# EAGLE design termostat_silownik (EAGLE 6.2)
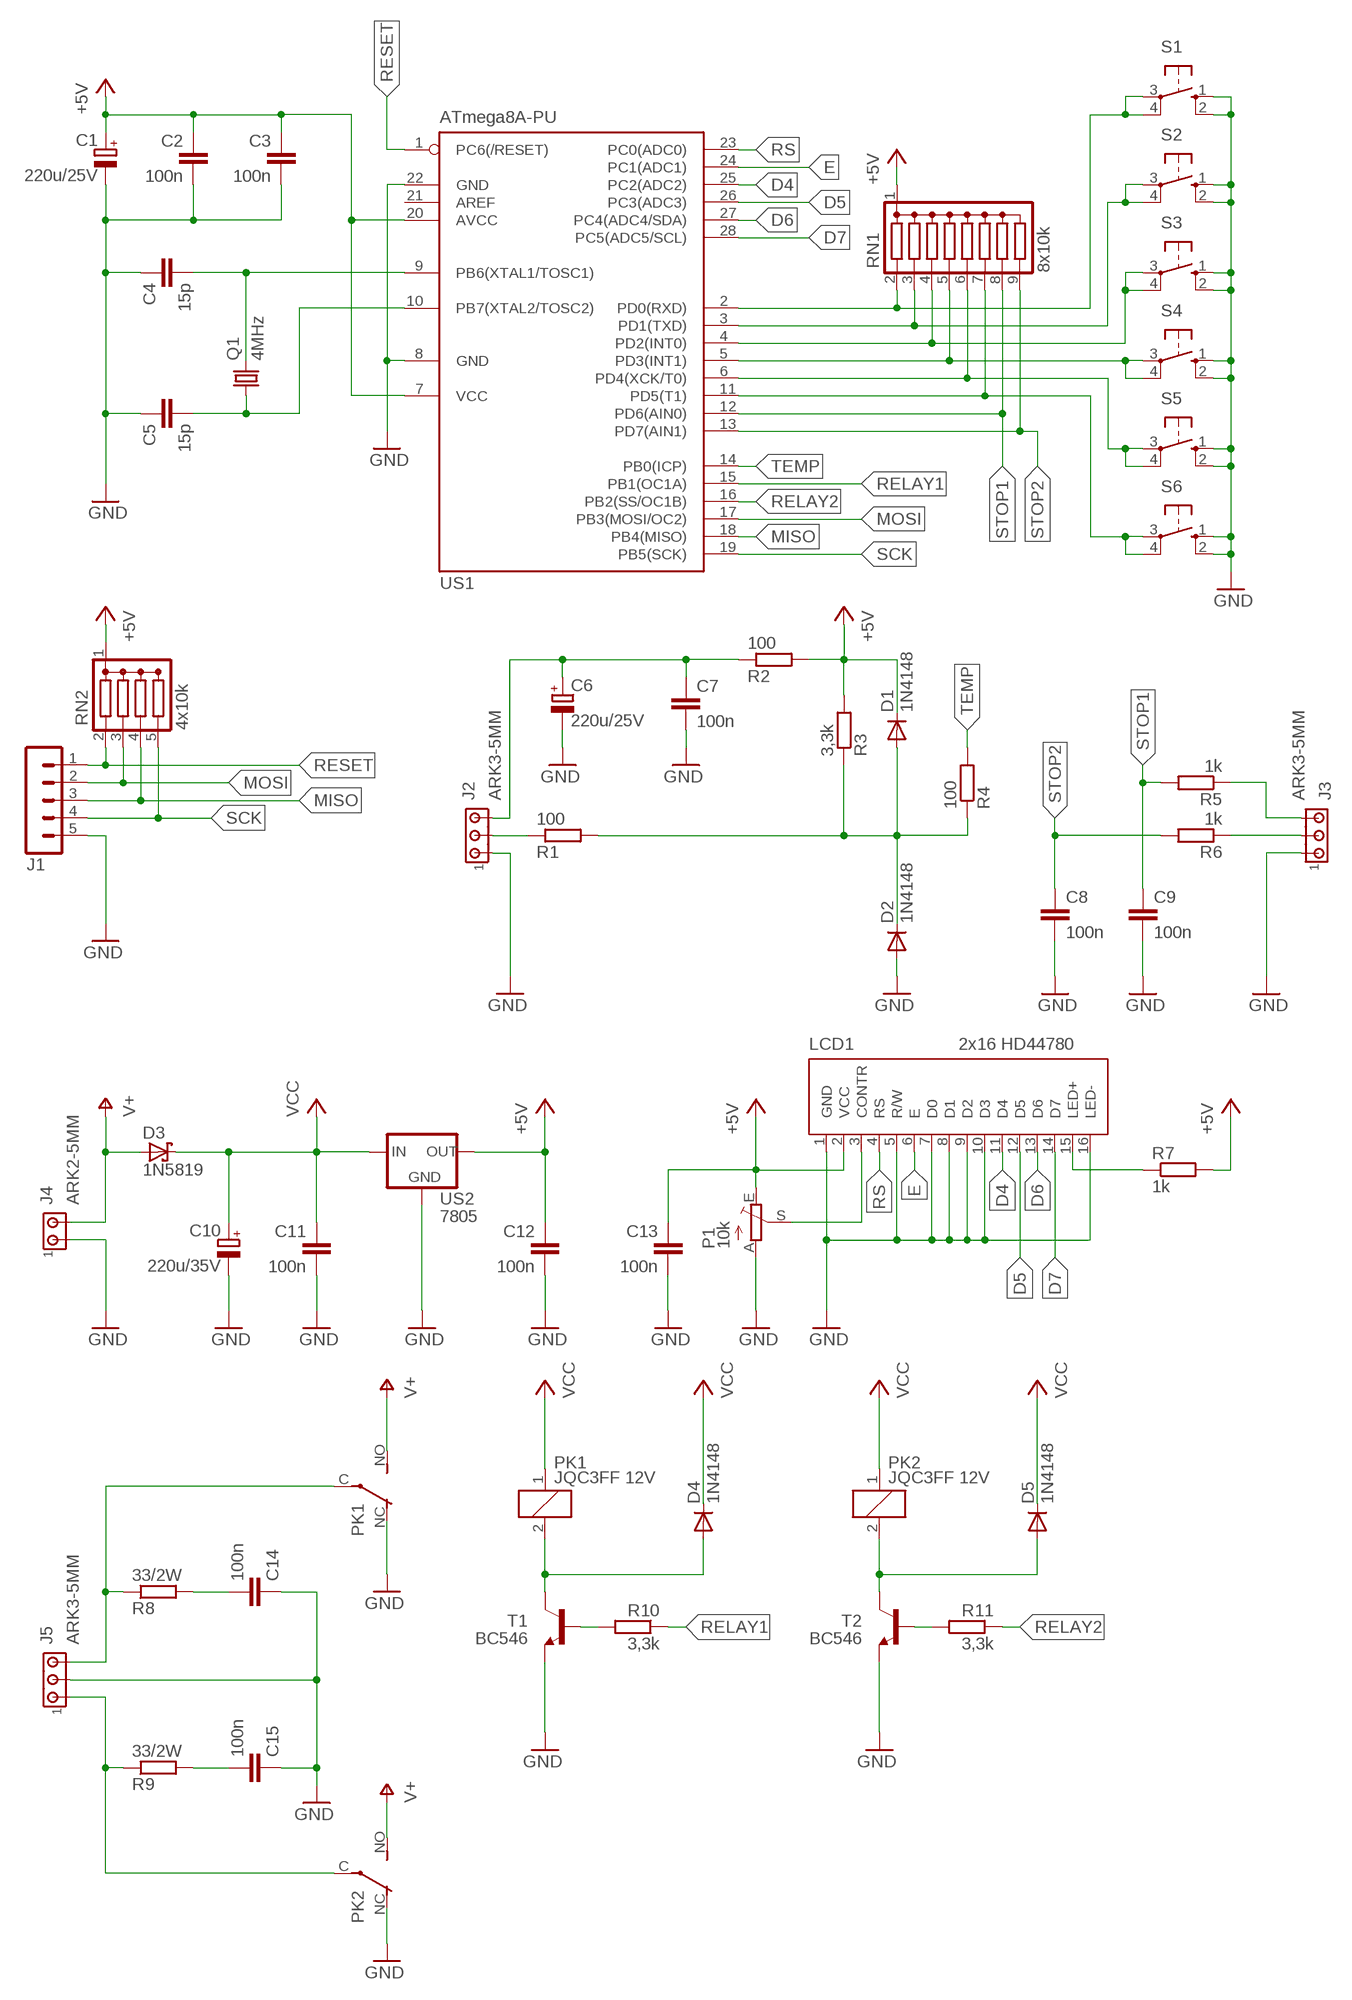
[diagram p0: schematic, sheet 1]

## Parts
C1  220u/25V  CPOL-EUE2.5-7  [E2,5-7]
C2  100n  C-EU050-025X075  [C050-025X075]
C3  100n  C-EU050-025X075  [C050-025X075]
C4  15p  C-EU050-025X075  [C050-025X075]
C5  15p  C-EU050-025X075  [C050-025X075]
C6  220u/25V  CPOL-EUE2.5-7  [E2,5-7]
C7  100n  C-EU050-025X075  [C050-025X075]
C8  100n  C-EU050-025X075  [C050-025X075]
C9  100n  C-EU050-025X075  [C050-025X075]
C10  220u/35V  CPOL-EUE3.5-8  [E3,5-8]
C11  100n  C-EU050-025X075  [C050-025X075]
C12  100n  C-EU050-025X075  [C050-025X075]
C13  100n  C-EU050-025X075  [C050-025X075]
C14  100n  C-EU050-025X075  [C050-025X075]
C15  100n  C-EU050-025X075  [C050-025X075]
D1  1N4148  BAT81  [DO34-7]
D2  1N4148  BAT81  [DO34-7]
D3  1N5819  SCHOTTKY-DIODEF126Z12  [F126Z12]
D4  1N4148  BAT81  [DO34-7]
D5  1N4148  BAT81  [DO34-7]
J1  MA05-1  [MA05-1]
J2  ARK3-5MM  [3PIN-5MM]
J3  ARK3-5MM  [3PIN-5MM]
J4  ARK2-5MM  [2PIN-5MM]
J5  ARK3-5MM  [3PIN-5MM]
LCD1  2x16 HD44780  LCD_2X16-NAD-ELEMENTAMI  [LCD_HD44780_2X16_NAD-ELEMENTAMI]
P1  10k  TRIM_EU-CA6V  [CA6V]
PK1  JQC3FF 12V  PK_POJED-JQC-3FG  [PK_POJED_JQC-3FG]
PK2  JQC3FF 12V  PK_POJED-JQC-3FG  [PK_POJED_JQC-3FG]
Q1  4MHz  CRYSTALHC49U-V  [HC49U-V]
R1  100  R-EU_0207/7  [0207/7]
R2  100  R-EU_0207/7  [0207/7]
R3  3,3k  R-EU_0207/7  [0207/7]
R4  100  R-EU_0207/7  [0207/7]
R5  1k  R-EU_0207/7  [0207/7]
R6  1k  R-EU_0207/7  [0207/7]
R7  1k  R-EU_0207/7  [0207/7]
R8  33/2W  R-EU_0411/15  [0411/15]
R9  33/2W  R-EU_0411/15  [0411/15]
R10  3,3k  R-EU_0207/7  [0207/7]
R11  3,3k  R-EU_0207/7  [0207/7]
RN1  8x10k  DRAB_REZ_1X8-SIL9  [RN-9]
RN2  4x10k  DRAB_REZ_1X4  [RN-5]
S1  10-XX  [B3F-10XX]
S2  10-XX  [B3F-10XX]
S3  10-XX  [B3F-10XX]
S4  10-XX  [B3F-10XX]
S5  10-XX  [B3F-10XX]
S6  10-XX  [B3F-10XX]
T1  BC546  BC546A  [TO92-EBC]
T2  BC546  BC546A  [TO92-EBC]
US1  ATmega8A-PU  MEGA8-P  [DIL28-3]
US2  7805  78XXS  [78XXS]

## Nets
+5V: C1.+ C2.1 C3.1 C12.1 C13.1 D1.C LCD1.2(VCC) P1.E R2.2 R3.2 R7.2 RN1.1(C) RN2.1(C) US1.7(VCC) US1.20(AVCC) US2.OUT
D4: LCD1.11(D4) US1.25(PC2(ADC2))
D5: LCD1.12(D5) US1.26(PC3(ADC3))
D6: LCD1.13(D6) US1.27(PC4(ADC4/SDA))
D7: LCD1.14(D7) US1.28(PC5(ADC5/SCL))
E: LCD1.6(E) US1.24(PC1(ADC1))
GND: C1.- C2.2 C3.2 C4.1 C5.1 C6.- C7.2 C8.2 C9.2 C10.- C11.2 C12.2 C13.2 C14.1 C15.1 D2.A J1.5 J2.P$1 J3.P$1 J4.P$1 J5.P$2 LCD1.1(GND) LCD1.5(R/W) LCD1.7(D0) LCD1.8(D1) LCD1.9(D2) LCD1.10(D3) LCD1.16(LED-) P1.A PK1.NC PK2.NC S1.1(S) S1.2(S1) S2.1(S) S2.2(S1) S3.1(S) S3.2(S1) S4.1(S) S4.2(S1) S5.1(S) S5.2(S1) S6.1(S) S6.2(S1) T1.E T2.E US1.8(GND) US1.22(GND) US2.GND
MISO: J1.3 RN2.4 US1.18(PB4(MISO))
MOSI: J1.2 RN2.3 US1.17(PB3(MOSI/OC2))
N$1: LCD1.3(CONTR) P1.S
N$2: R11.2 T2.B
N$3: C5.2 Q1.1 US1.10(PB7(XTAL2/TOSC2))
N$4: C4.2 Q1.2 US1.9(PB6(XTAL1/TOSC1))
N$5: RN1.2 S1.3(P) S1.4(P1) US1.2(PD0(RXD))
N$6: LCD1.15(LED+) R7.1
N$7: R10.2 T1.B
N$8: C15.2 R9.2
N$9: D4.A PK1.2 T1.C
N$10: RN1.3 S2.3(P) S2.4(P1) US1.3(PD1(TXD))
N$11: D5.A PK2.2 T2.C
N$12: C14.2 R8.2
N$13: RN1.4 S3.3(P) S3.4(P1) US1.4(PD2(INT0))
N$14: RN1.5 S4.3(P) S4.4(P1) US1.5(PD3(INT1))
N$15: RN1.6 S5.3(P) S5.4(P1) US1.6(PD4(XCK/T0))
N$16: RN1.7 S6.3(P) S6.4(P1) US1.11(PD5(T1))
N$17: J5.P$1 PK2.C(COM) R9.1
N$18: J5.P$3 PK1.C(COM) R8.1
N$19: C6.+ C7.1 J2.P$3 R2.1
N$20: J2.P$2 R1.1
N$21: D1.A D2.C R1.2 R3.1 R4.1
N$25: J3.P$2 R6.1
N$26: J3.P$3 R5.1
RELAY1: R10.1 US1.15(PB1(OC1A))
RELAY2: R11.1 US1.16(PB2(SS/OC1B))
RESET: J1.1 RN2.2 US1.1(PC6(/RESET))
RS: LCD1.4(RS) US1.23(PC0(ADC0))
SCK: J1.4 RN2.5 US1.19(PB5(SCK))
STOP1: C9.1 R5.2 RN1.8 US1.12(PD6(AIN0))
STOP2: C8.1 R6.2 RN1.9 US1.13(PD7(AIN1))
TEMP: R4.2 US1.14(PB0(ICP))
V+: D3.A J4.P$2 PK1.NO PK2.NO
VCC: C10.+ C11.1 D3.C D4.C D5.C PK1.1 PK2.1 US2.IN
Unconnected: US1.21(AREF)

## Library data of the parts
C1 C6 C10 = rcl:CPOL-EU: POLARIZED CAPACITOR, European symbol
C2-C5 C7-C9 C11-C15 = rcl:C-EU: CAPACITOR, European symbol
D1 D2 D4 D5 = diode:BAT81: DIODE
D3 = diode:SCHOTTKY-DIODE: Schottky Diode
J1 = zlacza_futrzak:MA05-1: PIN HEADER; OC_FARNELL: unknown; OC_NEWARK: unknown
J2 J3 J5 = zlacza_futrzak:ARK3: ARK 3 Raster 5mm i 3,5mm
J4 = zlacza_futrzak:ARK2: ARK 2
LCD1 = inne_futrzak:LCD_2X16
P1 = pot:TRIM_EU-: POTENTIOMETER
PK1 PK2 = inne_futrzak:PK_POJED
Q1 = crystal:CRYSTAL: CRYSTAL; OC_FARNELL: 1666969; OC_NEWARK: unknown
R1-R11 = rcl:R-EU_: RESISTOR, European symbol
RN1 = inne_futrzak:DRAB_REZ_1X8
RN2 = inne_futrzak:DRAB_REZ_1X4
S1-S6 = switch-omron:10-XX: OMRON SWITCH; MPN: B3F-1000; OC_FARNELL: 176432; OC_NEWARK: 36M3542
T1 T2 = transistor-npn:BC546*: NPN Transistor
US1 = atmel:MEGA8-P: MICROCONTROLLER 8 Kbytes FLASH, 1 kbytes SRAM, 512 bytes EEPROM, USART, 4-channel 10 bit ADC, 2-channel 8 bit ADC Pin compatible with Atmega48, ATMega88, ATMega168 Source: avr.lbr; OC_FARNELL: unknown; OC_NEWARK: unknown
US2 = v-reg:78XXS: VOLTAGE REGULATOR

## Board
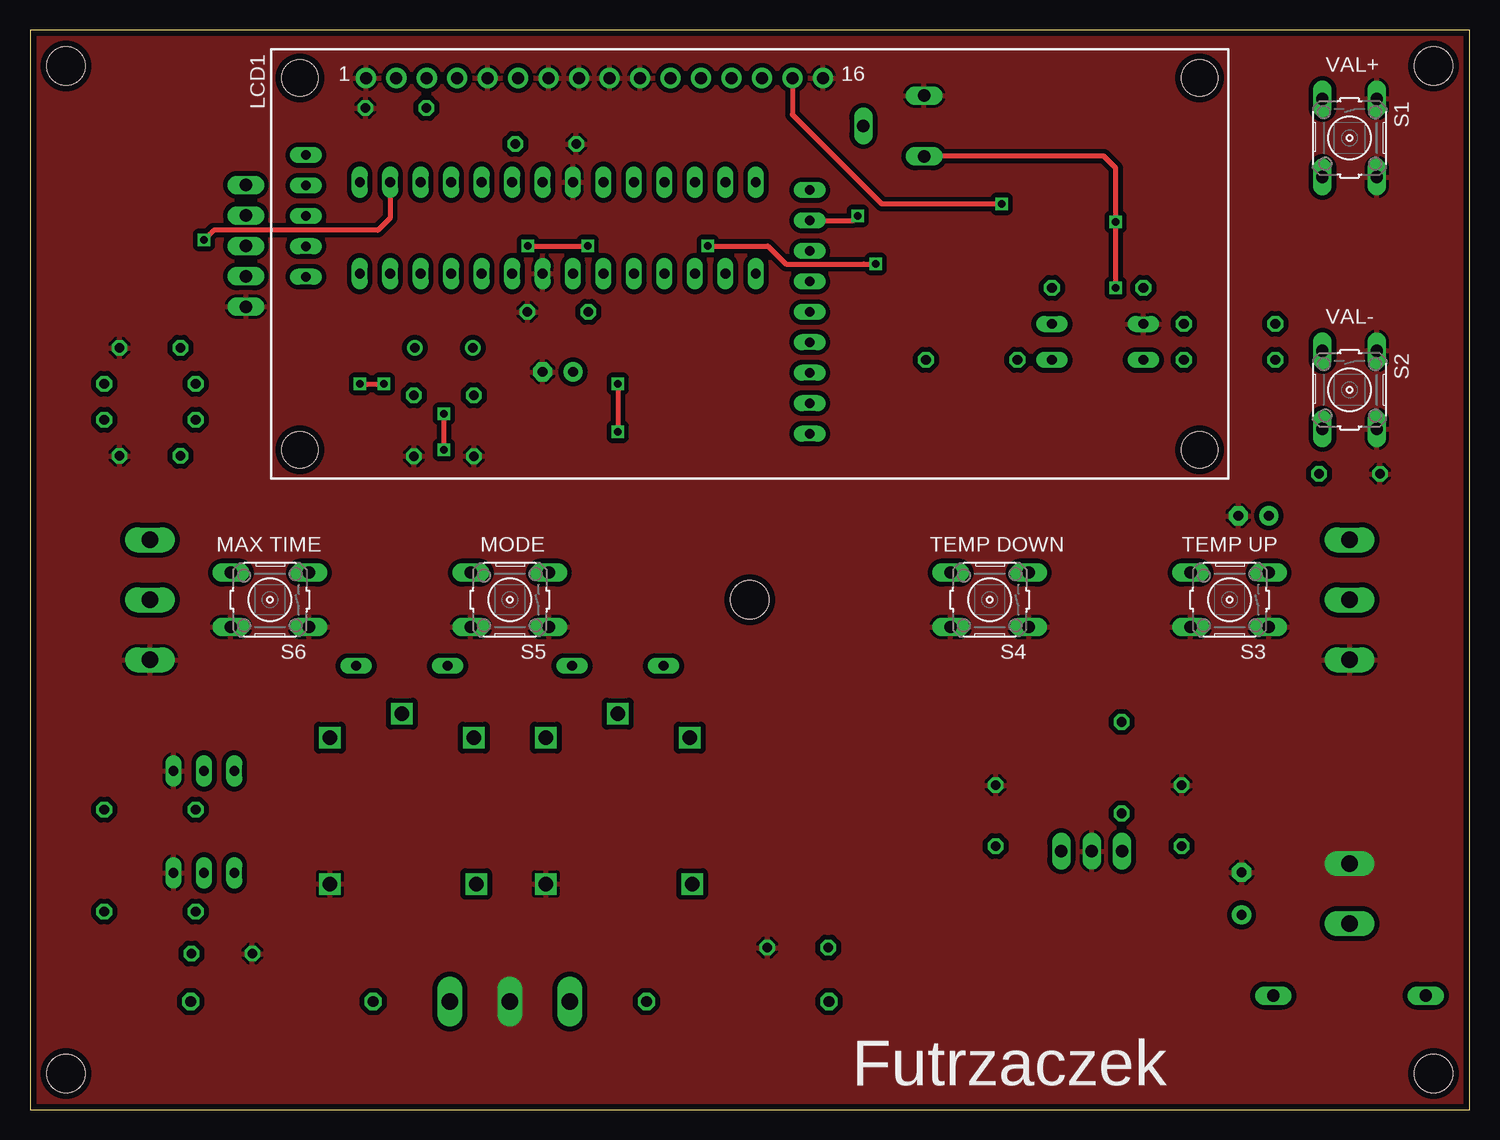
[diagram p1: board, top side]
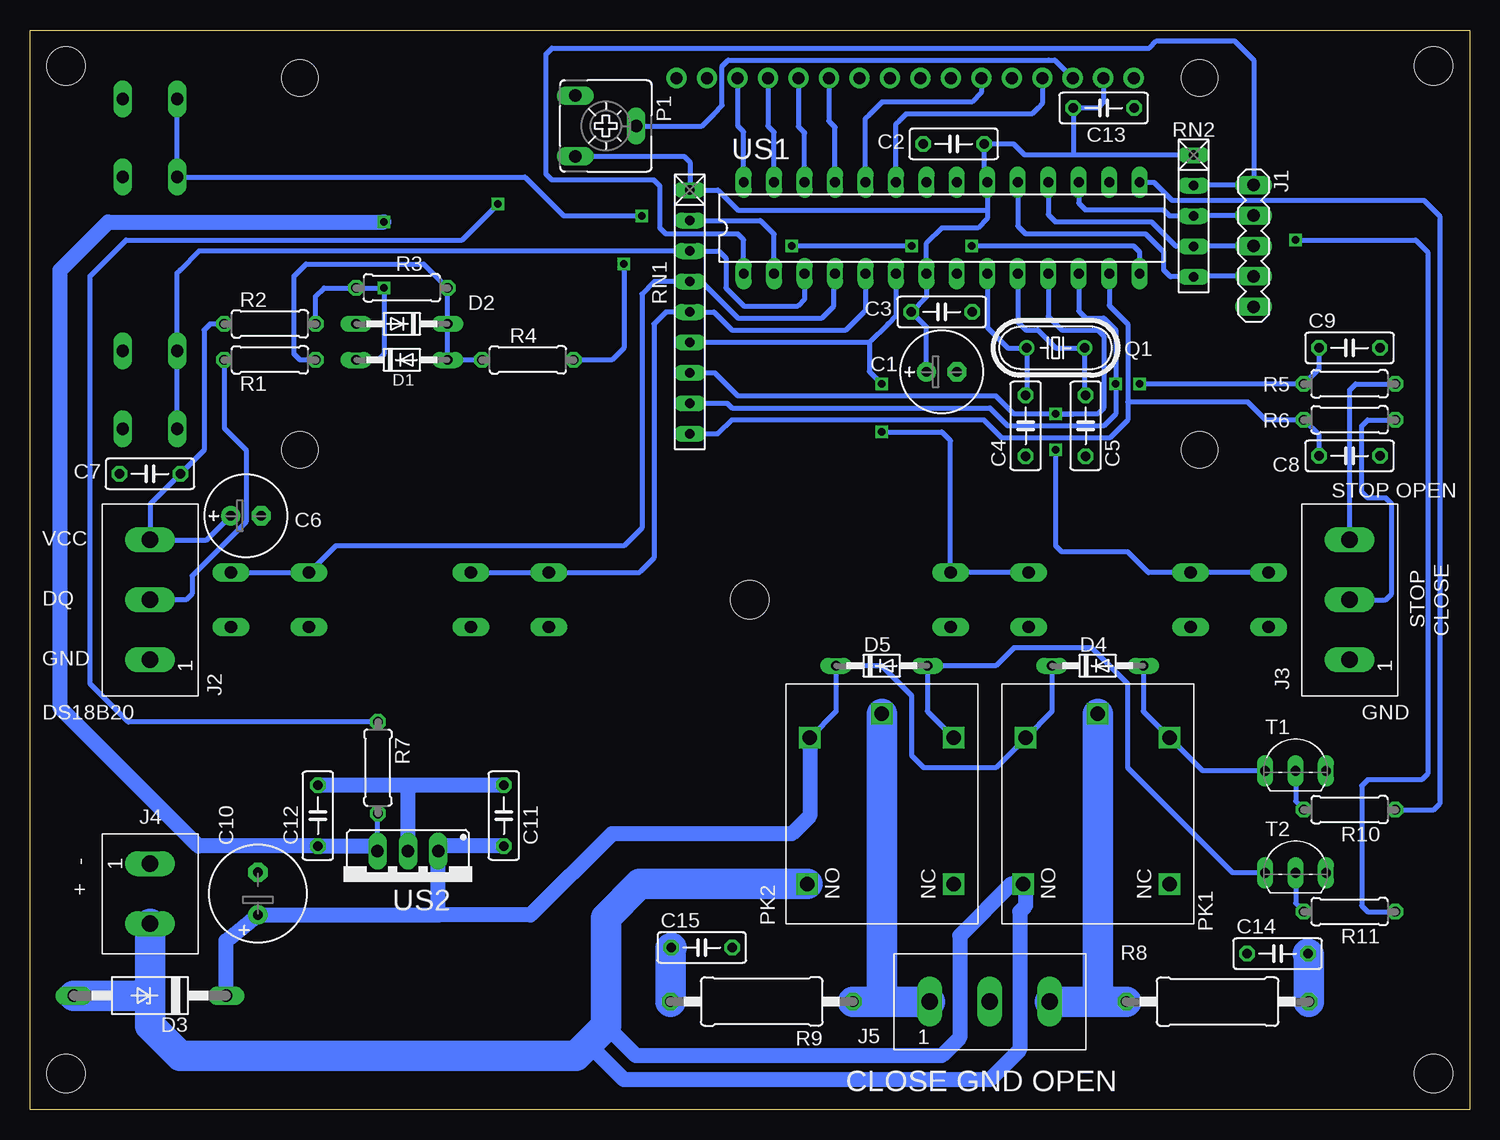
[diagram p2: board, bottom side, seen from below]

Size 120 x 90 mm. Coordinates in mm from the lower left corner, seen from the top.
Outline: 0,0 120,0 120,90 0,90 0,0
Copper layers (1*16): Top 0.035mm / dielectric 1.5mm / Bottom 0.035mm
Design rules: minimum track width 10mil, minimum drill 23mil, track to track 8mil, track to pad 8mil, pad to pad 8mil, via to via 8mil, smd to smd 8mil, copper to edge 20mil, drill to drill 8mil, minimum pad ring 10mil, minimum via ring 8mil, stop-mask expansion 4mil, vias tented up to drill 0mil, thermal gap 10mil
Holes 3.2 mm at 3,87 117,87 3,3 117,3 60,42.5

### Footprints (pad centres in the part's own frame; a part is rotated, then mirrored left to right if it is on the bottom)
E2,5-7 = drill 0.813 pad 1.6: + -1.27,0 | drill 0.813 pad 1.6 octagon: - 1.27,0
C050-025X075 = drill 0.813 octagon: 1 -2.54,0; 2 2.54,0
E3,5-8 = drill 0.813 pad 1.6: + -1.778,0 | drill 0.813 pad 1.6 octagon: - 1.778,0
DO34-7 = drill 0.813 long: A 3.81,0; C -3.81,0
F126Z12 = drill 1.016 long: A 6.35,0; C -6.35,0
MA05-1 = drill 1.016 long: 1 -5.08,0; 2 -2.54,0; 3 0,0; 4 2.54,0; 5 5.08,0
3PIN-5MM = drill 1.4 long: P$1 -5,0; P$2 0,0; P$3 5,0
2PIN-5MM = drill 1.4 long: P$1 -2.5,0; P$2 2.5,0
LCD_HD44780_2X16_NAD-ELEMENTAMI = drill 1 pad 1.676: 1 -32,15.5; 2 -29.46,15.5; 3 -26.92,15.5; 4 -24.38,15.5; 5 -21.84,15.5; 6 -19.3,15.5; 7 -16.76,15.5; 8 -14.22,15.5; 9 -11.68,15.5; 10 -9.14,15.5; 11 -6.6,15.5; 12 -4.06,15.5; 13 -1.52,15.5; 14 1.02,15.5; 15 3.56,15.5; 16 6.1,15.5 | hole 3: -37.5,-15.5; 37.5,-15.5; -37.5,15.5; 37.5,15.5
CA6V = drill 1.016 long: A -2.54,-2.54; E 2.54,-2.54; S 0,2.54
PK_POJED_JQC-3FG = drill 1.2 square: 1 5.5,6; 2 5.5,-6; C 7.5,0; NC -6.7,-6; NO -6.7,6.2
HC49U-V = drill 0.813: 1 -2.413,0; 2 2.413,0
0207/7 = drill 0.813 octagon: 1 -3.81,0; 2 3.81,0
0411/15 = drill 0.914 octagon: 1 -7.62,0; 2 7.62,0
RN-9 = drill 0.813 long: 1 -10.16,0; 2 -7.62,0; 3 -5.08,0; 4 -2.54,0; 5 0,0; 6 2.54,0; 7 5.08,0; 8 7.62,0; 9 10.16,0
RN-5 = drill 0.813 long: 1 -5.08,0; 2 -2.54,0; 3 0,0; 4 2.54,0; 5 5.08,0
B3F-10XX = drill 1.016 long: 1 -3.251,2.261; 2 3.251,2.261; 3 -3.251,-2.261; 4 3.251,-2.261
TO92-EBC = drill 0.813 long: B 0,-1.27; C -2.54,-1.27; E 2.54,-1.27
DIL28-3 = drill 0.813 long: 1 -16.51,-3.81; 2 -13.97,-3.81; 3 -11.43,-3.81; 4 -8.89,-3.81; 5 -6.35,-3.81; 6 -3.81,-3.81; 7 -1.27,-3.81; 8 1.27,-3.81; 9 3.81,-3.81; 10 6.35,-3.81; 11 8.89,-3.81; 12 11.43,-3.81; 13 13.97,-3.81; 14 16.51,-3.81; 15 16.51,3.81; 16 13.97,3.81; 17 11.43,3.81; 18 8.89,3.81; 19 6.35,3.81; 20 3.81,3.81; 21 1.27,3.81; 22 -1.27,3.81; 23 -3.81,3.81; 24 -6.35,3.81; 25 -8.89,3.81; 26 -11.43,3.81; 27 -13.97,3.81; 28 -16.51,3.81
78XXS = drill 1.016 long: GND 0,-2.54; IN -2.54,-2.54; OUT 2.54,-2.54

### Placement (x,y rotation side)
C1  44,61.5 0 bottom
C2  43,80.5 180 bottom
C3  44,66.5 0 bottom
C4  37,57 90 bottom
C5  32,57 90 bottom
C6  102,49.5 0 bottom
C7  110,53 180 bottom
C8  10,54.5 0 bottom
C9  10,63.5 0 bottom
C10  101,18 90 bottom
C11  80.5,24.5 90 bottom
C12  96,24.5 90 bottom
C13  30.5,83.5 0 bottom
C14  16,13 0 bottom
C15  64,13.5 180 bottom
D1  89,62.5 0 bottom
D2  89,65.5 180 bottom
D3  110,9.5 180 bottom
D4  31,37 0 bottom
D5  49,37 0 bottom
J1  18,72 270 bottom
J2  110,42.5 90 bottom
J3  10,42.5 90 bottom
J4  110,18 270 bottom
J5  40,9 0 bottom
LCD1  60,70.5 0 top
P1  72,82 270 bottom
PK1  31,25.5 90 bottom
PK2  49,25.5 90 bottom
Q1  34.5,63.5 180 bottom
R1  100,62.5 0 bottom
R2  100,65.5 0 bottom
R3  89,68.5 180 bottom
R4  78.5,62.5 0 bottom
R5  10,60.5 180 bottom
R6  10,57.5 180 bottom
R7  91,28.5 270 bottom
R8  21,9 0 bottom
R9  59,9 180 bottom
R10  10,25 180 bottom
R11  10,16.5 180 bottom
RN1  65,66.5 270 bottom
RN2  23,74.5 270 bottom
S1  110,81 270 top
S2  110,60 270 top
S3  100,42.5 180 top
S4  80,42.5 180 top
S5  40,42.5 180 top
S6  20,42.5 180 top
T1  14.5,29.5 0 bottom
T2  14.5,21 0 bottom
US1  44,73.5 0 bottom
US2  88.5,19 180 bottom

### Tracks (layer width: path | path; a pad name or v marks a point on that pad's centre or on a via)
+5V  (via drill 0.6)
  Top 0.406: v90.5,68.5 v90.5,74 90.5,78.5 89.5,79.5 74.58,79.5 P1.E
  Bottom 0.406: 40.19,75 US1.20 40.46,77.58 C2.1 38,80.5 37.08,79.58 33,79.58 | 40.19,75 40.19,74.31 41,73.5 44,73.5 45.27,72.23 US1.7 45.27,67.77 C3.1 45.27,65.23 C1.+ | RN2.1 33,79.58 | 33,79.58 33.04,79.62 C13.1 31,83.5 30.54,83.96 LCD1.2 | 40.19,75 61,75 62.66,76.66 RN1.1 65,79 65.46,79.46 P1.E | D1.C 91,62.5 90.5,63 v90.5,68.5 R3.2 95.5,68.5 96.19,67.81 R2.2 | US2.OUT 91.04,24.65 R7.2
  Bottom 1.27: v90.5,74 113.5,74 117.5,70 117.5,33.5 105.96,21.96 C12.1 91.04,21.96 US2.OUT
D4
  Bottom 0.406: US1.25 52.89,81.89 53,82 53.4,82.4 LCD1.11
D5
  Bottom 0.406: US1.26 55.43,81.43 55.94,81.94 LCD1.12
D6
  Bottom 0.406: US1.27 57.97,81.47 58.48,81.98 LCD1.13
D7
  Bottom 0.406: US1.28 60.51,81.51 61,82 61.02,82.02 LCD1.14
E
  Bottom 0.406: LCD1.6 40.7,84.8 41.5,84 49,84 50,83 50.35,82.65 US1.24
GND
  Bottom 1.27: C11.2 88.5,27.04 | 88.5,27.04 C12.2 | US2.GND 88.5,27.04
  pour Top (isolate 0.406): 0,0 120,0 120,90 0,90
  pour Top (no thermals): 38.5,12 41.5,12 41.5,6 38.5,6
  pour Top (no thermals): 107.5,22 112.5,22 112.5,19 107.5,19
MISO
  Bottom 0.406: J1.3 22.96,72 RN2.4 24.46,71.96 26.5,74 34.5,74 35.11,74.61 US1.18
MOSI
  Bottom 0.406: J1.2 22.96,74.54 RN2.3 25,74.5 25.5,75 32,75 32.57,75.57 US1.17
N$1
  Bottom 0.406: P1.S 64,82 63,83 62.3,83.7 62.3,87 61.8,87.5 35.08,87.5 34.58,87.5 LCD1.3
N$2
  Bottom 0.406: T2.B 14.5,17.19 R11.2
N$3
  Bottom 0.406: US1.10 37.65,65.65 37,65 36,65 34.5,63.5 Q1.1 32.09,59.63 C5.2
N$4
  Bottom 0.406: US1.9 40.19,65.19 38.5,63.5 Q1.2 36.91,59.63 C4.2
N$5  (via drill 0.6)
  Top 0.406: RN1.2 68.62,74.12 v69,74.5
  Bottom 0.406: RN1.2 59.12,74.12 58,73 57.97,72.97 US1.2 | v69,74.5 75.5,74.5 78.5,77.5 78.75,77.75 S1.4 S1.3
N$6  (via drill 0.6)
  Top 0.406: v81,75.5 71,75.5 63.56,82.94 LCD1.15
  Bottom 0.406: R7.1 111.81,32.31 115,35.5 115,69.5 112,72.5 84,72.5 v81,75.5
N$7
  Bottom 0.406: T1.B 14.5,25.69 R10.2
N$8
  Bottom 2.54: R9.2 66.62,13.42 C15.2
N$9
  Bottom 0.406: T1.C 22.23,28.23 PK1.2 27.19,33.19 D4.A
N$10
  Bottom 0.406: US1.3 55.43,67.57 56,67 60.5,67 62,68.5 62,71 62.58,71.58 RN1.3 105.92,71.58 107.5,70 107.74,69.76 S2.3 S2.4
N$11
  Bottom 0.406: PK2.2 45.19,33.19 D5.A 39.5,37 38,38.5 31.5,38.5 28.5,35.5 28.5,28.5 19.73,19.73 T2.C
N$12
  Bottom 2.54: R8.2 13.38,12.92 C14.2
N$13
  Bottom 0.406: US1.4 53,69.58 53,67 54,66 61,66 63,68 64.04,69.04 RN1.4 67.96,69.04 69,68 69,48.5 70.5,47 94.51,47 S3.4 S3.3
N$14
  Bottom 0.406: US1.5 50.35,66.65 50.5,66.5 52,65 61.5,65 63,66.5 RN1.5 67,66.5 68,65.5 68,46 69,45 69.24,44.76 S4.4 S4.3
N$15  (via drill 0.6)
  Top 0.406: v49,60.5 v49,56.5
  Bottom 0.406: RN1.6 50.04,63.96 | 50.04,63.96 48.5,65.5 47.81,66.19 US1.6 | S5.4 S5.3 43.25,55.75 43.5,56 44,56.5 v49,56.5 | 50.04,63.96 50.04,61.54 v49,60.5
N$16  (via drill 0.6)
  Top 0.406: v34.5,55 v34.5,58
  Bottom 0.406: US1.11 35.11,66.11 34,65 31,65 30.5,64.5 30.5,58.5 31,58 33,58 | 33,58 v34.5,58 | v34.5,58 38,58 39.5,59.5 61,59.5 62.25,60.75 | 62.25,60.75 62.5,61 | RN1.7 62.92,61.42 62.25,60.75 | S6.4 S6.3 26.76,44.76 27.5,45.5 28.5,46.5 34,46.5 34.5,47 v34.5,55 | v34.5,58 33,58
N$17
  Bottom 2.54: J5.P$1 49,9 | 49,9 R9.1 | PK2.C 49,9
N$18
  Bottom 2.54: R8.1 31,9 | 31,9 J5.P$3 | PK1.C 31,9
N$19
  Bottom 0.406: C6.+ 105.27,47.5 J2.P$3 110,50.46 C7.1 105.5,54.96 105.5,65 105,65.5 R2.1
N$20
  Bottom 0.406: R1.1 103.81,56.81 102,55 102,49 106.5,44.5 106.5,43 107,42.5 J2.P$2
N$21
  Bottom 0.406: R4.1 D1.A D2.C R3.1 87.19,70.5 97,70.5 98,69.5 98,63 97.5,62.5 R1.2
N$25
  Bottom 0.406: J3.P$2 7,42.5 6.5,43 6.5,50.5 7,51 8.5,51 9,51.5 9,57 8.5,57.5 R6.1
N$26
  Bottom 0.406: J3.P$3 10,60 9.5,60.5 R5.1
RELAY1
  Bottom 0.406: US1.15 26.31,77.31 24.8,75.8 3.8,75.8 2.5,74.5 2.5,25.5 3,25 R10.1
RELAY2  (via drill 0.6)
  Top 0.406: US1.16 30.03,74.33 29,73.3 15.3,73.3 v14.5,72.5
  Bottom 0.406: v14.5,72.5 4.5,72.5 3.5,71.5 3.5,28 4,27.5 8.5,27.5 9,27 9,17 8.5,16.5 R11.1
RESET
  Bottom 0.406: RN2.2 22.96,77.08 J1.1 18,87.5 19,88.5 19.6,89.1 26.1,89.1 26.7,88.5 76.5,88.5 77,88 77,78 76.5,77.5 68,77.5 67.5,77 67.5,73.5 67,73 61,73 60.51,72.51 US1.1
RS
  Bottom 0.406: LCD1.4 35.62,83.88 36,83.5 36.5,83 47,83 47.5,82.5 47.81,82.19 US1.23
SCK
  Bottom 0.406: J1.4 22.96,69.46 RN2.5 23.92,69.42 24.92,69.42 25.5,70 25.5,71.5 26.5,72.5 27,73 37,73 37.5,73.5 37.65,73.65 US1.19
STOP1  (via drill 0.6)
  Top 0.406: v27.5,60.5 v29.5,60.5
  Bottom 0.406: US1.12 32.57,66.57 32,66 30.5,66 29.5,65 v29.5,60.5 29.5,58 30.5,57 38.5,57 40,58.5 61.5,58.5 61.88,58.88 RN1.8 | v27.5,60.5 R5.2 12.54,61.77 C9.1
STOP2
  Bottom 0.406: US1.13 30.03,67.03 28.5,65.5 28.5,59 | 28.5,59 28.5,57.5 30,56 39,56 40.5,57.5 61.5,57.5 62.66,56.34 RN1.9 | C8.1 12.54,56.23 R6.2 17,57.5 18.5,59 28.5,59
TEMP  (via drill 0.6)
  Top 0.406: v41.5,72 v46.5,72 | v56.5,72 61.5,72 62.5,71 63,70.5 69.5,70.5 v70.5,70.5
  Bottom 0.406: US1.14 27.49,71.49 28,72 v41.5,72 | v46.5,72 v56.5,72 | v70.5,70.5 70.5,63.5 71.5,62.5 R4.2
V+
  Bottom 1.27: 73.5,5.5 70.5,2.5 40,2.5 37.5,5 37.5,16.5 37,17 37,18.5 | PK1.NO 38.2,18.8 42.5,14.5 42.5,6 44,4.5 69.5,4.5 72,7
  Bottom 2.54: PK2.NO 69.2,18.8 72,16 72,7 73.5,5.5 74.5,4.5 107.5,4.5 110,7 110,9.5 | 110,9.5 J4.P$2 | D3.A 110,9.5
VCC
  Bottom 0.406: D4.C 34.81,33.19 PK1.1 39.5,28.5 45.5,28.5 46.5,29.5 46.5,34.5 49,37 D5.C 52.81,33.19 PK2.1
  Bottom 1.27: D3.C 103.65,14.08 C10.+ 85.96,16.22 | 85.96,16.22 US2.IN 85.96,21.96 C11.1 | PK2.1 55,24.5 56.5,23 71.5,23 78.28,16.22 85.96,16.22

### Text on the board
tPlace: VAL+ | VAL- | MAX TIME | MODE | TEMP DOWN | TEMP UP | Futrzaczek
bPlace: STOP OPEN | VCC | CLOSE | STOP | DQ | GND | GND | DS18B20 | + - | CLOSE GND OPEN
